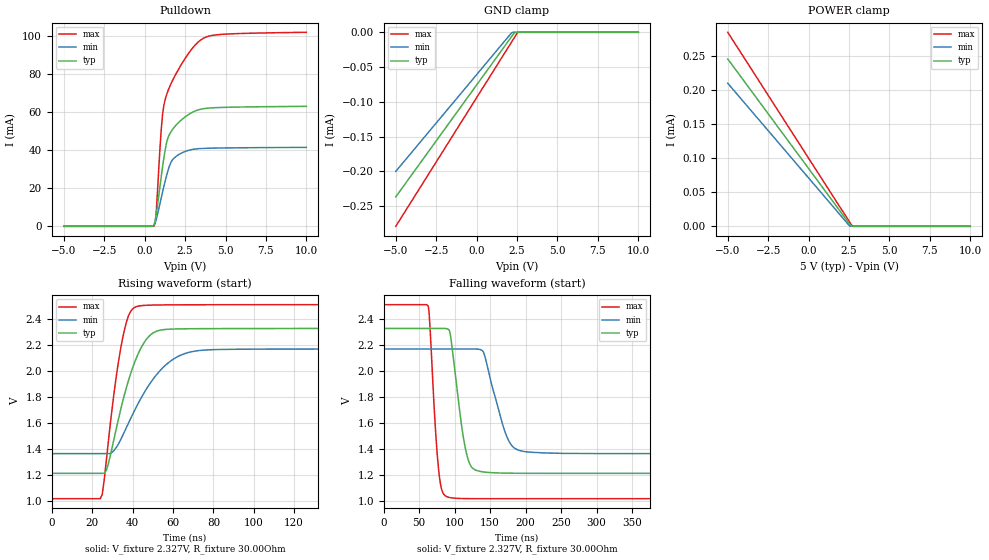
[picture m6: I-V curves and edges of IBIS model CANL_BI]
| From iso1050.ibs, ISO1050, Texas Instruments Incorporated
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|   CANL Model
[Model]   CANL_BI
Model_type   I/O_open_drain
| Signals   CANL
Vinh  = 0.9V
Vinl  = 0.5V
Rref  = 30Ohm   |Note: 60 Ohm differential load;
Vref  = 2.327V   |tr, tf measured in single ended configuration"
Vmeas = 2.3VV
| variable   typ   min   max
C_comp   2.6707pF   3.4333pF   2.7489pF
|   typ   min   max
[Temperature Range]   40   125   -55
[Voltage Range]   5.0V   4.75V   5.25V
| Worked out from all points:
|   slope of the pulldown table from 0 to 0.75 V, typ, clamps not added: 90.4 ohm
|   falling waveform, V_fixture 2.327V, R_fixture 30.00Ohm: 20-80 % time 15.9ns typ, 24.2ns min, 9.6ns max; typ from 2.33 V to 1.21 V
|   rising waveform, V_fixture 2.327V, R_fixture 30.00Ohm: 20-80 % time 11.8ns typ, 18.2ns min, 7.54ns max; typ from 1.21 V to 2.33 V
[Pulldown]
|   Voltage   I(typ)   I(min)   I(max)
-5V       0A         0A         0A
577.9mV   754.8uA    647.5uA    112.9uA
653.3mV   3.056mA    1.944mA    1.804mA
728.6mV   6.976mA    4.049mA    9.102mA
1.03V     26.42mA    15.12mA    51.47mA
1.106V    31.12mA    17.94mA    58.73mA
1.256V    39.57mA    23.35mA    66.18mA
1.482V    47.36mA    30.37mA    72.03mA
1.784V    51.54mA    35.53mA    77.6mA
3.367V    61.28mA    40.79mA    97.21mA
4.648V    62.41mA    41.12mA    100.7mA
10V       63.01mA    41.46mA    101.9mA
[GND Clamp]
|   Voltage   I(typ)   I(min)   I(max)
-5V       -236.6uA   -200uA     -279uA
2.161V    -6.249uA   -790.7nA   -14.08uA
2.387V    0A         0A         -5.711uA
2.538V    0A         0A         -134.8nA
10V       0A         0A         0A
[POWER Clamp]
|   Voltage   I(typ)   I(min)   I(max)
-5V       245.8uA    210.2uA    285.1uA
2.538V    3.451uA    487.8nA    6.325uA
2.688V    0A         0A         748.2nA
10V       0A         0A         0A
[Ramp]
R_load = 30.00Ohm
|   typ   min   max
dV/dt_r   668.994mV/11.771ns  483.258mV/18.176ns  895.798mV/7.543ns
dV/dt_f   668.994mV/15.903ns  483.258mV/24.125ns  895.798mV/9.601ns
[Falling Waveform]
V_fixture = 2.327V
V_fixture_min = 2.169V
V_fixture_max = 2.510V
R_fixture = 30.00Ohm
|   Time   V(typ)   V(min)   V(max)
0s        2.327V     2.169V     2.51V
63ns      2.327V     2.169V     2.496V
77ns      2.327V     2.169V     1.265V
88ns      2.326V     2.169V     1.035V
94ns      2.279V     2.169V     1.025V
115ns     1.409V     2.169V     1.018V
128ns     1.242V     2.169V     1.017V
141ns     1.222V     2.14V      1.017V
188ns     1.213V     1.395V     1.017V
500ns     1.212V     1.364V     1.017V
[Rising Waveform]
V_fixture = 2.327V
V_fixture_min = 2.169V
V_fixture_max = 2.510V
R_fixture = 30.00Ohm
|   Time   V(typ)   V(min)   V(max)
0s        1.212V     1.364V     1.017V
25ns      1.212V     1.364V     1.049V
28ns      1.283V     1.364V     1.452V
35ns      1.757V     1.499V     2.244V
39ns      1.976V     1.632V     2.456V
43ns      2.139V     1.756V     2.499V
49ns      2.279V     1.912V     2.507V
58ns      2.321V     2.066V     2.508V
77ns      2.326V     2.162V     2.509V
500ns     2.327V     2.169V     2.51V
